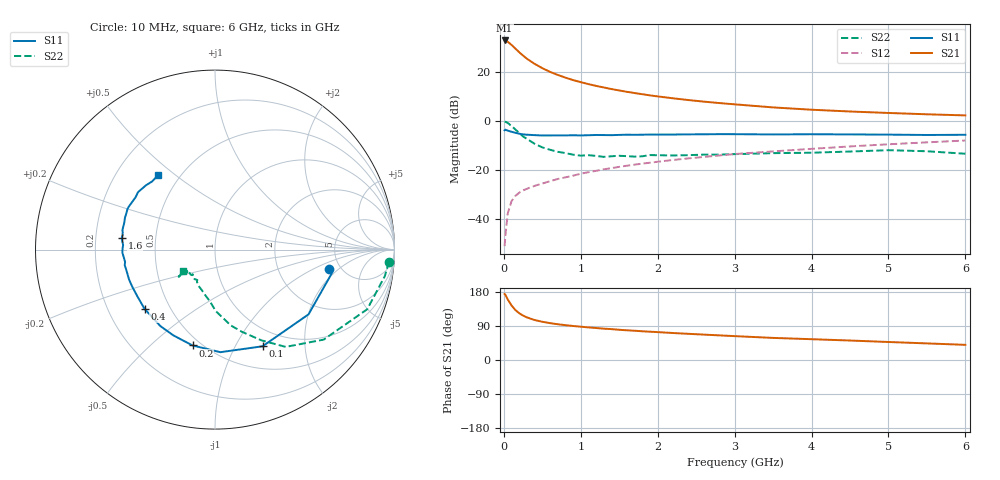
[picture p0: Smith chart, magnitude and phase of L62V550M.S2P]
!  INFINEON TECHNOLOGIES Small Signal Semiconductors
! BFR380L3 , Si-NPN RF-Transistor in TSLP-3-1
!  Vce=2.5 V,  Ic=50 mA
! Common Emitter S-Parameters:  07. March 2005
#  GHz  S  MA  R  50
! f  S11  S21  S12  S22
! GHz  Mag  Ang  Mag  Ang  Mag  Ang  Mag  Ang
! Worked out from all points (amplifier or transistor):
!   36 points, 10 MHz to 6 GHz, reference 50 ohm
!   highest |S21| = 32.8 dB at 10 MHz (marker M1)
!   |S21| within 3 dB of that: start of sweep to 139.7 MHz
!   unconditionally stable (mu >= 1): 1.545 GHz to 4.851 GHz
!   at 250 MHz: K = 0.49, MSG = 27.5 dB, |S12| = -28.3 dB
!   at 1.4 GHz: K = 0.99, MSG = 16.1 dB, |S12| = -19.3 dB
!   at 6 GHz: K = 0.98, MSG = 5.1 dB, |S12| = -8.0 dB
!   S11 on the Smith chart (normalised r, x): 10 MHz: 4.03, -1.49; 100 MHz: 0.77, -1.30; 200 MHz: 0.45, -0.69; 400 MHz: 0.36, -0.32; 1.6 GHz: 0.31, +0.06; 6 GHz: 0.38, +0.43
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0.01  0.6437 -9.7  43.62 174.1  0.0028 79.2  0.9707 -4.0
0.02  0.6632 -11.7  43.01 172.0  0.0046 86.6  0.9581 -8.8
0.05  0.6338 -34.7  41.08 160.0  0.0129 77.0  0.9109 -21.4
0.1  0.6003 -63.8  35.46 143.9  0.0231 65.7  0.7864 -39.6
0.15  0.5724 -87.0  29.79 131.8  0.0296 59.3  0.6701 -54.0
0.2  0.5485 -103.2  25.07 123.4  0.0344 56.9  0.568 -62.9
0.25  0.5312 -115.9  21.47 117.2  0.0384 53.8  0.4823 -71.8
0.3  0.5235 -125.6  18.53 112.4  0.0414 54.1  0.4309 -78.3
0.4  0.5129 -139.9  14.54 105.5  0.0475 54.4  0.3418 -89.4
0.5  0.5048 -149.2  11.9 100.9  0.0529 55.8  0.2889 -95.7
0.6  0.5053 -155.9  9.995 97.3  0.0591 57.5  0.2585 -102.4
0.7  0.507 -160.9  8.664 94.4  0.0655 59.5  0.235 -108.8
0.9  0.5103 -170.3  6.793 89.8  0.0766 62.1  0.2052 -119.4
1.1  0.511 -175.6  5.62 86.0  0.0902 64.0  0.2002 -124.7
1.3  0.5147 178.9  4.799 82.7  0.1034 64.4  0.1849 -132.4
1.6  0.5238 172.7  3.914 78.4  0.1222 65.8  0.1913 -139.3
2.2  0.5273 163.4  2.889 71.2  0.1601 66.1  0.1975 -141.2
2.8  0.5375 155.0  2.311 65.0  0.1974 65.8  0.2056 -146.8
3.5  0.5299 146.7  1.884 58.3  0.2392 63.6  0.2202 -145.0
4.5  0.5304 140.6  1.556 51.4  0.3018 61.8  0.2377 -144.0
5.5  0.5167 132.7  1.364 43.8  0.3658 57.8  0.2407 -143.6
6  0.5215 127.6  1.295 40.0  0.3986 55.6  0.2143 -146.2
